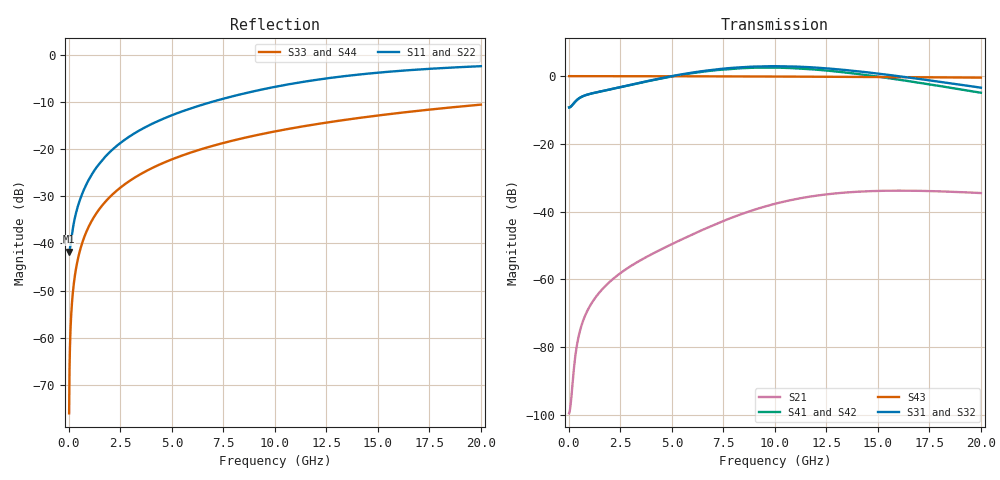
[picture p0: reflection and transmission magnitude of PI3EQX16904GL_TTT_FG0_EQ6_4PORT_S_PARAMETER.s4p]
! NPort=4 DATA=2000 NOISE=0 GROUPDELAY=0 COMPLEX_DATAFORMAT=POLAR
! NumOfBlock=1 NumOfParam=0
! .MODEL Smodel S TSTONEFILE=PI3EQX16904GL_TTT_FG0_EQ6_4PORT_S_PARAMETER.s4p TYPE=S
!  -- The above .MODEL line can be used for the S element in the netlist.
! The s parameter is extracted from the linear redriver, it is not bi-directional; only s(4,1)s(4,2) and s(3,1)s(3,2)
! should be the insertion loss
!Port definition:
!Port1 = input+
!Port2 = input-
!Port3 = output+
!Port4 = output-
# Hz S MA R  50
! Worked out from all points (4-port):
!   2000 points, 10 MHz to 20 GHz, reference 50 ohm
!   strongest paths, dB at 10 MHz, 5.01 GHz, 10.01 GHz, 15.01 GHz, 20 GHz:
!     S31: -9.2, 0.0, 2.9, 0.8, -3.4
!     S32: -9.2, 0.0, 2.8, 0.5, -3.7
!     S43: 0.0, 0.0, -0.1, -0.3, -0.4
!     S41: -9.2, -0.1, 2.5, -0.2, -4.9
!     S42: -9.2, -0.1, 2.4, -0.4, -5.2
!     S21: -99.6, -49.6, -37.7, -33.9, -34.5
!   lowest |S11| = -41.7 dB at 10 MHz (marker M1), VSWR 1.02, Z = 49.2 - j0.0603 ohm
!   |S11| at or under -10 dB: start of sweep to 6.872 GHz
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1e7  0.008182 -175.7  1.05e-05 7.8  0 0.0  0 0.0
     1.05e-05 7.8  0.008182 -175.7  0 0.0  0 0.0
     0.3452 0.7  0.3452 -179.3  0.0001571 -90.0  1 -0.0
     0.3452 -179.3  0.3452 0.7  1 -0.0  0.0001571 -90.0
3.8e8  0.02256 -119.7  0.0001024 118.3  0 0.0  0 0.0
       0.0001024 118.3  0.02256 -119.7  0 0.0  0 0.0
       0.4422 13.9  0.4422 -166.2  0.005969 -90.4  1 -0.3
       0.4422 -166.8  0.4422 13.1  1 -0.3  0.005969 -90.4
1.6e9  0.07608 -102.8  0.0007037 109.1  0 0.0  0 0.0
       0.0007034 109.1  0.07608 -102.8  0 0.0  0 0.0
       0.6002 6.2  0.6004 -174.1  0.02512 -91.5  0.9997 -1.4
       0.5994 -176.7  0.5997 3.0  0.9997 -1.4  0.02512 -91.5
5.84e9  0.2688 -104.6  0.004405 101.4  0 0.0  0 0.0
        0.004372 101.7  0.2688 -104.6  0 0.0  0 0.0
        1.11 -35.7  1.1 143.4  0.09132 -95.4  0.9955 -5.2
        1.091 133.9  1.081 -47.0  0.9955 -5.2  0.09132 -95.4
9.61e9  0.4432 -111.8  0.0122 71.1  0 0.0  0 0.0
        0.0121 72.0  0.443 -111.8  0 0.0  0 0.0
        1.401 -96.2  1.379 82.8  0.1491 -98.9  0.9879 -8.6
        1.339 67.0  1.318 -114.0  0.9879 -8.6  0.1491 -98.9
1.37e10  0.6104 -122.4  0.0195 22.0  0 0.0  0 0.0
         0.01939 23.4  0.6101 -122.3  0 0.0  0 0.0
         1.208 -162.7  1.183 16.2  0.21 -102.6  0.9759 -12.1
         1.107 -5.9  1.083 173.0  0.9759 -12.1  0.21 -102.6
2e10  0.7649 -136.4  0.01877 -36.1  0 0.0  0 0.0
      0.01878 -34.0  0.7652 -136.3  0 0.0  0 0.0
      0.6757 114.8  0.6557 -66.2  0.2986 -108.1  0.9506 -17.4
      0.5689 -97.2  0.5521 81.9  0.9506 -17.4  0.2986 -108.1
